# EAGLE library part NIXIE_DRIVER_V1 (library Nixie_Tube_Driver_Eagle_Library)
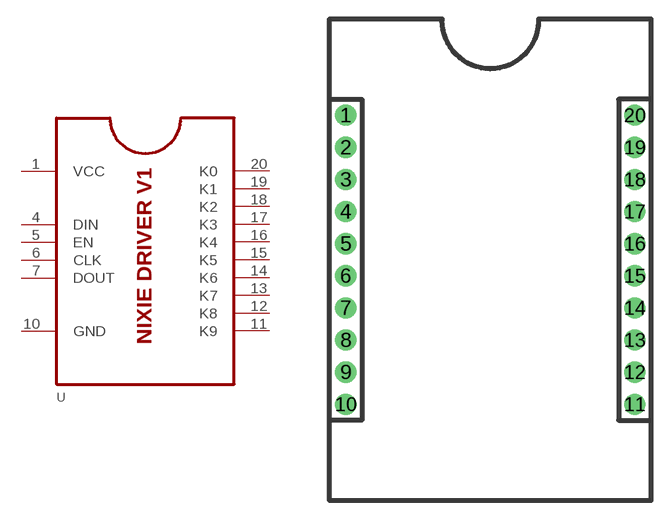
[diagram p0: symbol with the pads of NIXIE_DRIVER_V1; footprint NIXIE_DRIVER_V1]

Designator prefix -

## NIXIE_DRIVER_V1  [NIXIE_DRIVER_V1]
1  VCC  pwr
4  DIN  pas
5  EN  pas
6  CLK  pas
7  DOUT  pas
10  GND  pwr
11  K9  pas
12  K8  pas
13  K7  pas
14  K6  pas
15  K5  pas
16  K4  pas
17  K3  pas
18  K2  pas
19  K1  pas
20  K0  pas

## Footprint NIXIE_DRIVER_V1 (pad centres in mm)
drill 1 pad 1.676: 1 -11.43,11.43; 2 -11.43,8.89; 3 -11.43,6.35; 4 -11.43,3.81; 5 -11.43,1.27; 6 -11.43,-1.27; 7 -11.43,-3.81; 8 -11.43,-6.35; 9 -11.43,-8.89; 10 -11.43,-11.43; 11 11.43,-11.43; 12 11.43,-8.89; 13 11.43,-6.35; 14 11.43,-3.81; 15 11.43,-1.27; 16 11.43,1.27; 17 11.43,3.81; 18 11.43,6.35; 19 11.43,8.89; 20 11.43,11.43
